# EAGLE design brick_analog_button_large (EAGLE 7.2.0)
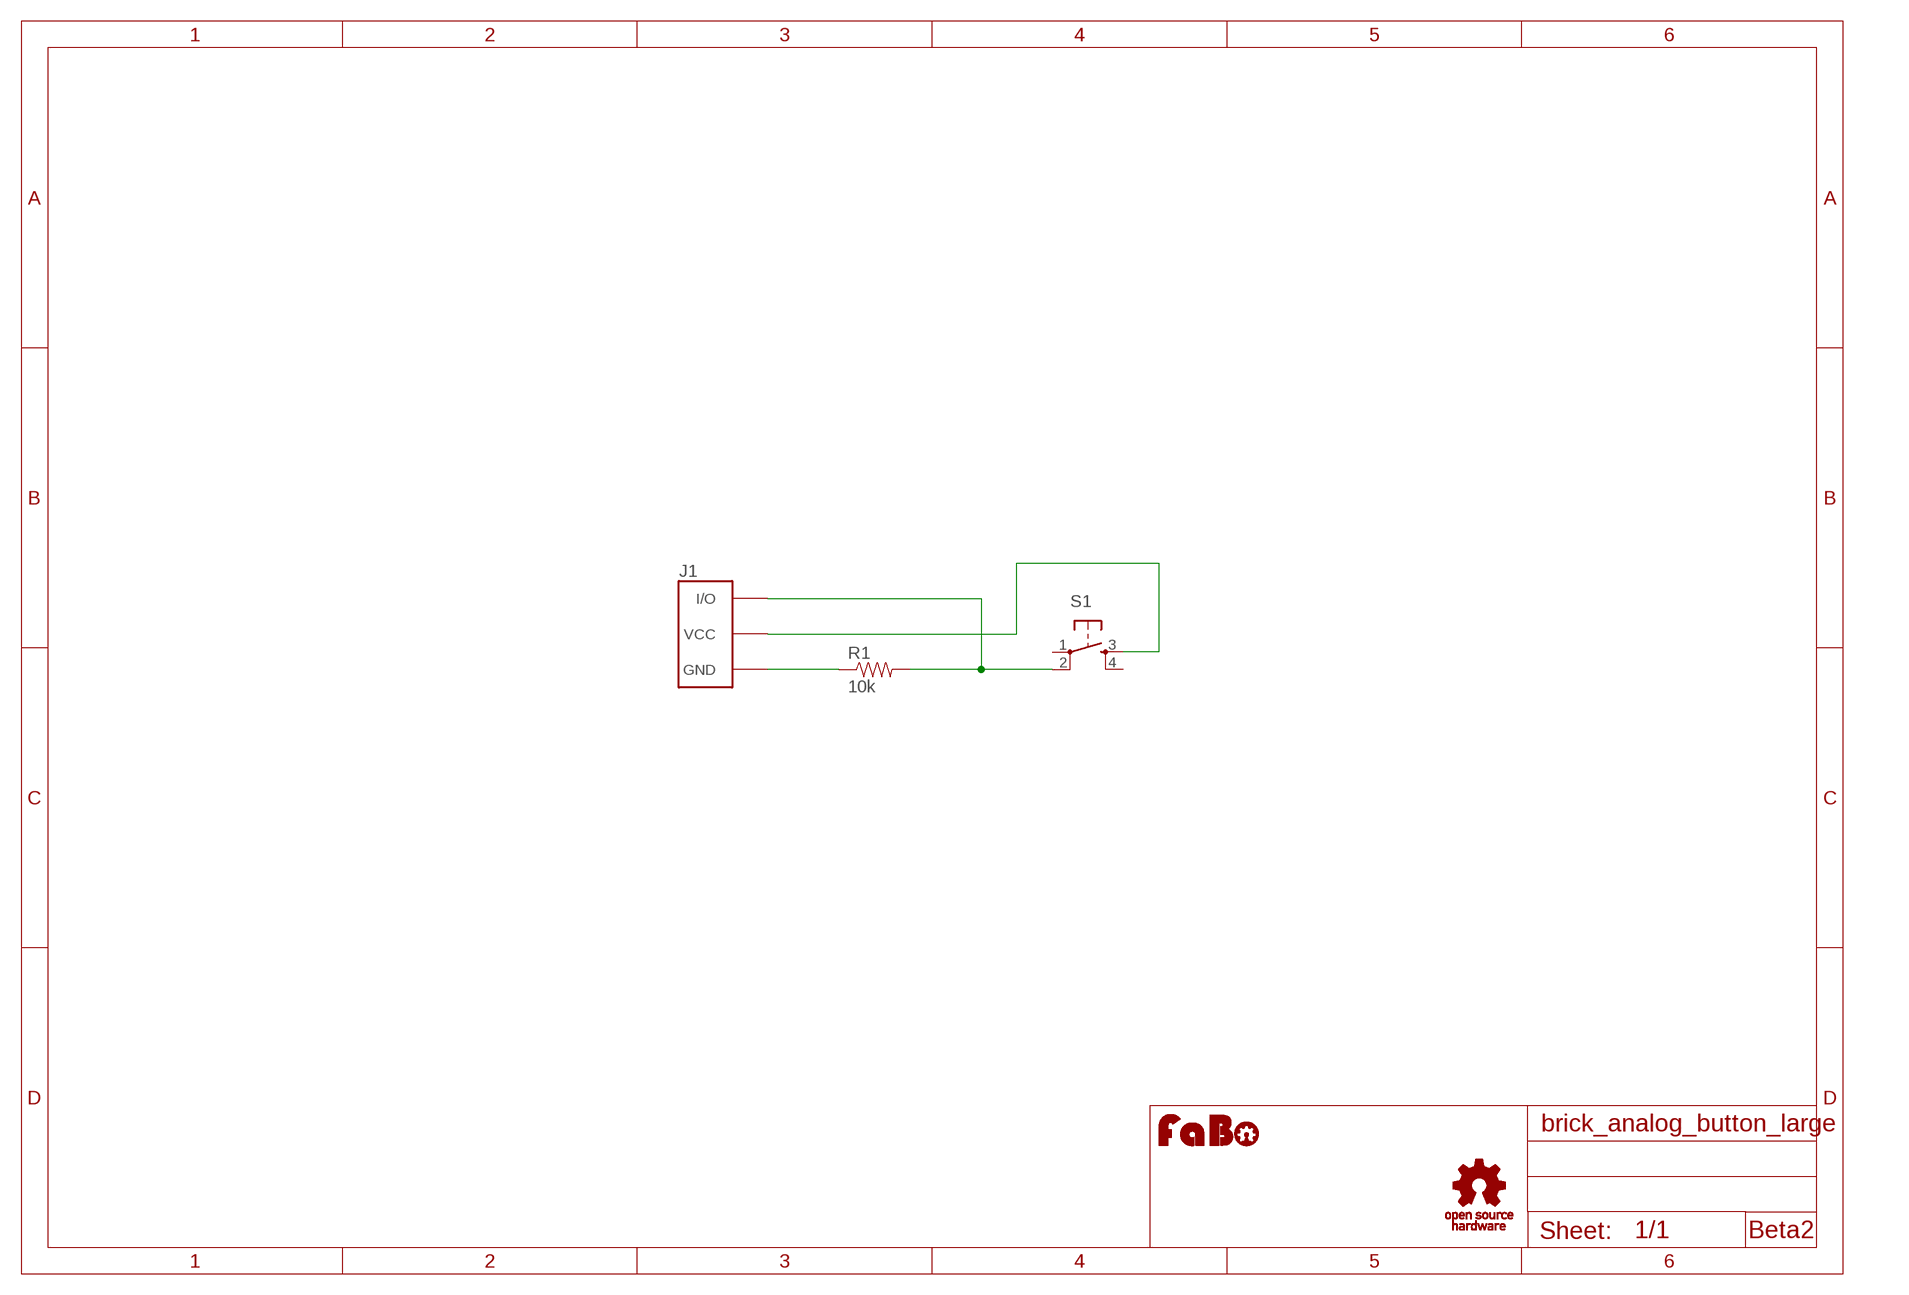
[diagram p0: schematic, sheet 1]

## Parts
J1  BRICK_3PIN  [BRICK_3PIN]
R1  10k  RES-PTH-REGULAR  [RES-AXL-REGULAR]
S1  SWITCH-TACT-12MM  [1273HA-160G-G]
U$2  LOGO_FABO-S  [LOGO_FABO_S]
U$3  LOGO_OSHW_T-S  [LOGO_OSHW_T_S]

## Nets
GND: J1.GND R1.P$1
N$1: J1.VCC S1.3
N$4: J1.IN/OUT(I/O) R1.P$2 S1.2
Unconnected: S1.1 S1.4

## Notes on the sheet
- Beta2

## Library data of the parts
J1 = gclue:BRICK_3PIN: FaBo Brick 3pin
R1 = gclue:RES
S1 = gclue:SWITCH-TACT
U$2 = FaBo:LOGO_FABO
U$3 = gclue:LOGO_OSHW_T

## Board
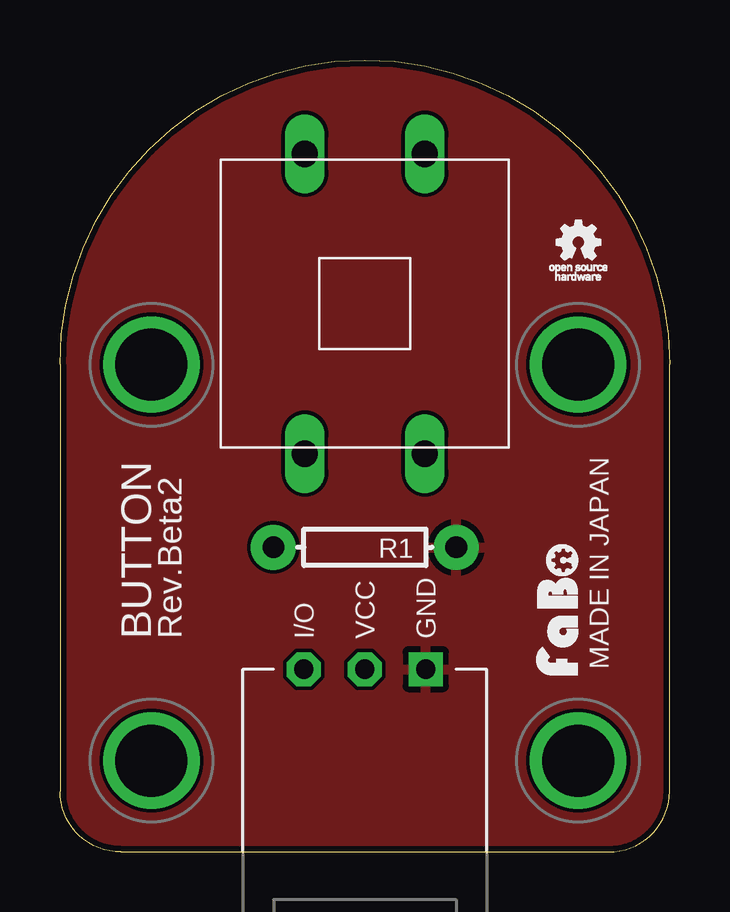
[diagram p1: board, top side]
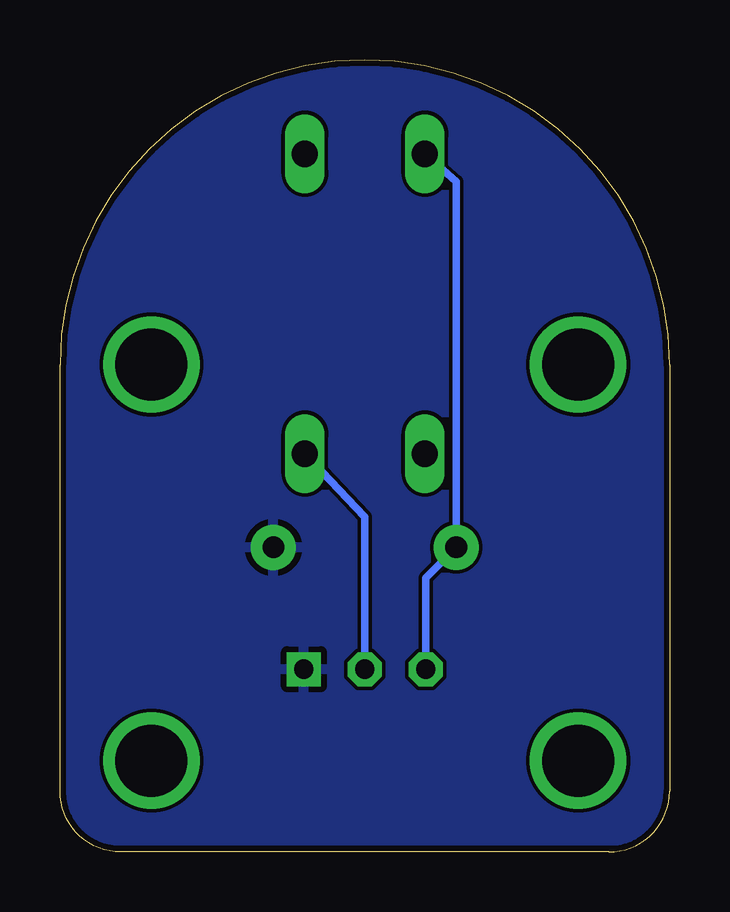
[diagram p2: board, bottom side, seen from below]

Size 25.4 x 33.02 mm. Coordinates in mm from the lower left corner, seen from the top.
Copper layers (1*16): Top 0.035mm / dielectric 1.5mm / Bottom 0.035mm
Design rules "Elecrow_2-layer_eagle_rule": minimum track width 6mil, minimum drill 12mil, track to track 6mil, track to pad 6mil, pad to pad 6mil, via to via 6mil, smd to smd 0mil, copper to edge 10mil, drill to drill 10mil, minimum pad ring 10mil, minimum via ring 6mil, stop-mask expansion 2mil, vias tented up to drill 100mil, thermal gap 10mil

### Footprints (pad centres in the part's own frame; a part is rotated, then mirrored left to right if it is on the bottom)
BRICK_3PIN = drill 0.8 pad 1.422 square: GND 2.54,-8.89 | drill 0.8 pad 1.422 octagon: IN/OUT -2.54,-8.89; VCC 0,-8.89 | drill 3 pad 3.81: P$5 -8.89,3.81; P$6 8.89,3.81; P$7 -8.89,-12.7; P$8 8.89,-12.7
RES-AXL-REGULAR = drill 0.9 pad 1.88: P$1 -3.81,0; P$2 3.81,0
1273HA-160G-G = drill 1.1 long: 1 -6.25,2.5; 2 6.25,2.5; 3 -6.25,-2.5; 4 6.25,-2.5

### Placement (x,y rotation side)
J1  12.7,16.51 0 top
R1  12.7,12.7 180 top
S1  12.7,22.86 90 top
U$2  21.59,10.16 90 top
U$3  21.59,25.4 0 top

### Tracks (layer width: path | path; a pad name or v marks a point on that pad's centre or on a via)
GND
  pour Bottom: -1.27,-1.27 26.67,-1.27 26.67,34.29 -1.27,34.29
  pour Top: -1.27,-1.27 26.67,-1.27 26.67,34.29 -1.27,34.29
N$1
  Bottom 0.305: J1.VCC 12.7,13.97 S1.3
N$4
  Bottom 0.305: J1.IN/OUT 10.16,11.43 R1.P$2 8.89,27.94 S1.2

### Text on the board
tPlace: BUTTON | Rev.Beta2 | MADE IN JAPAN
